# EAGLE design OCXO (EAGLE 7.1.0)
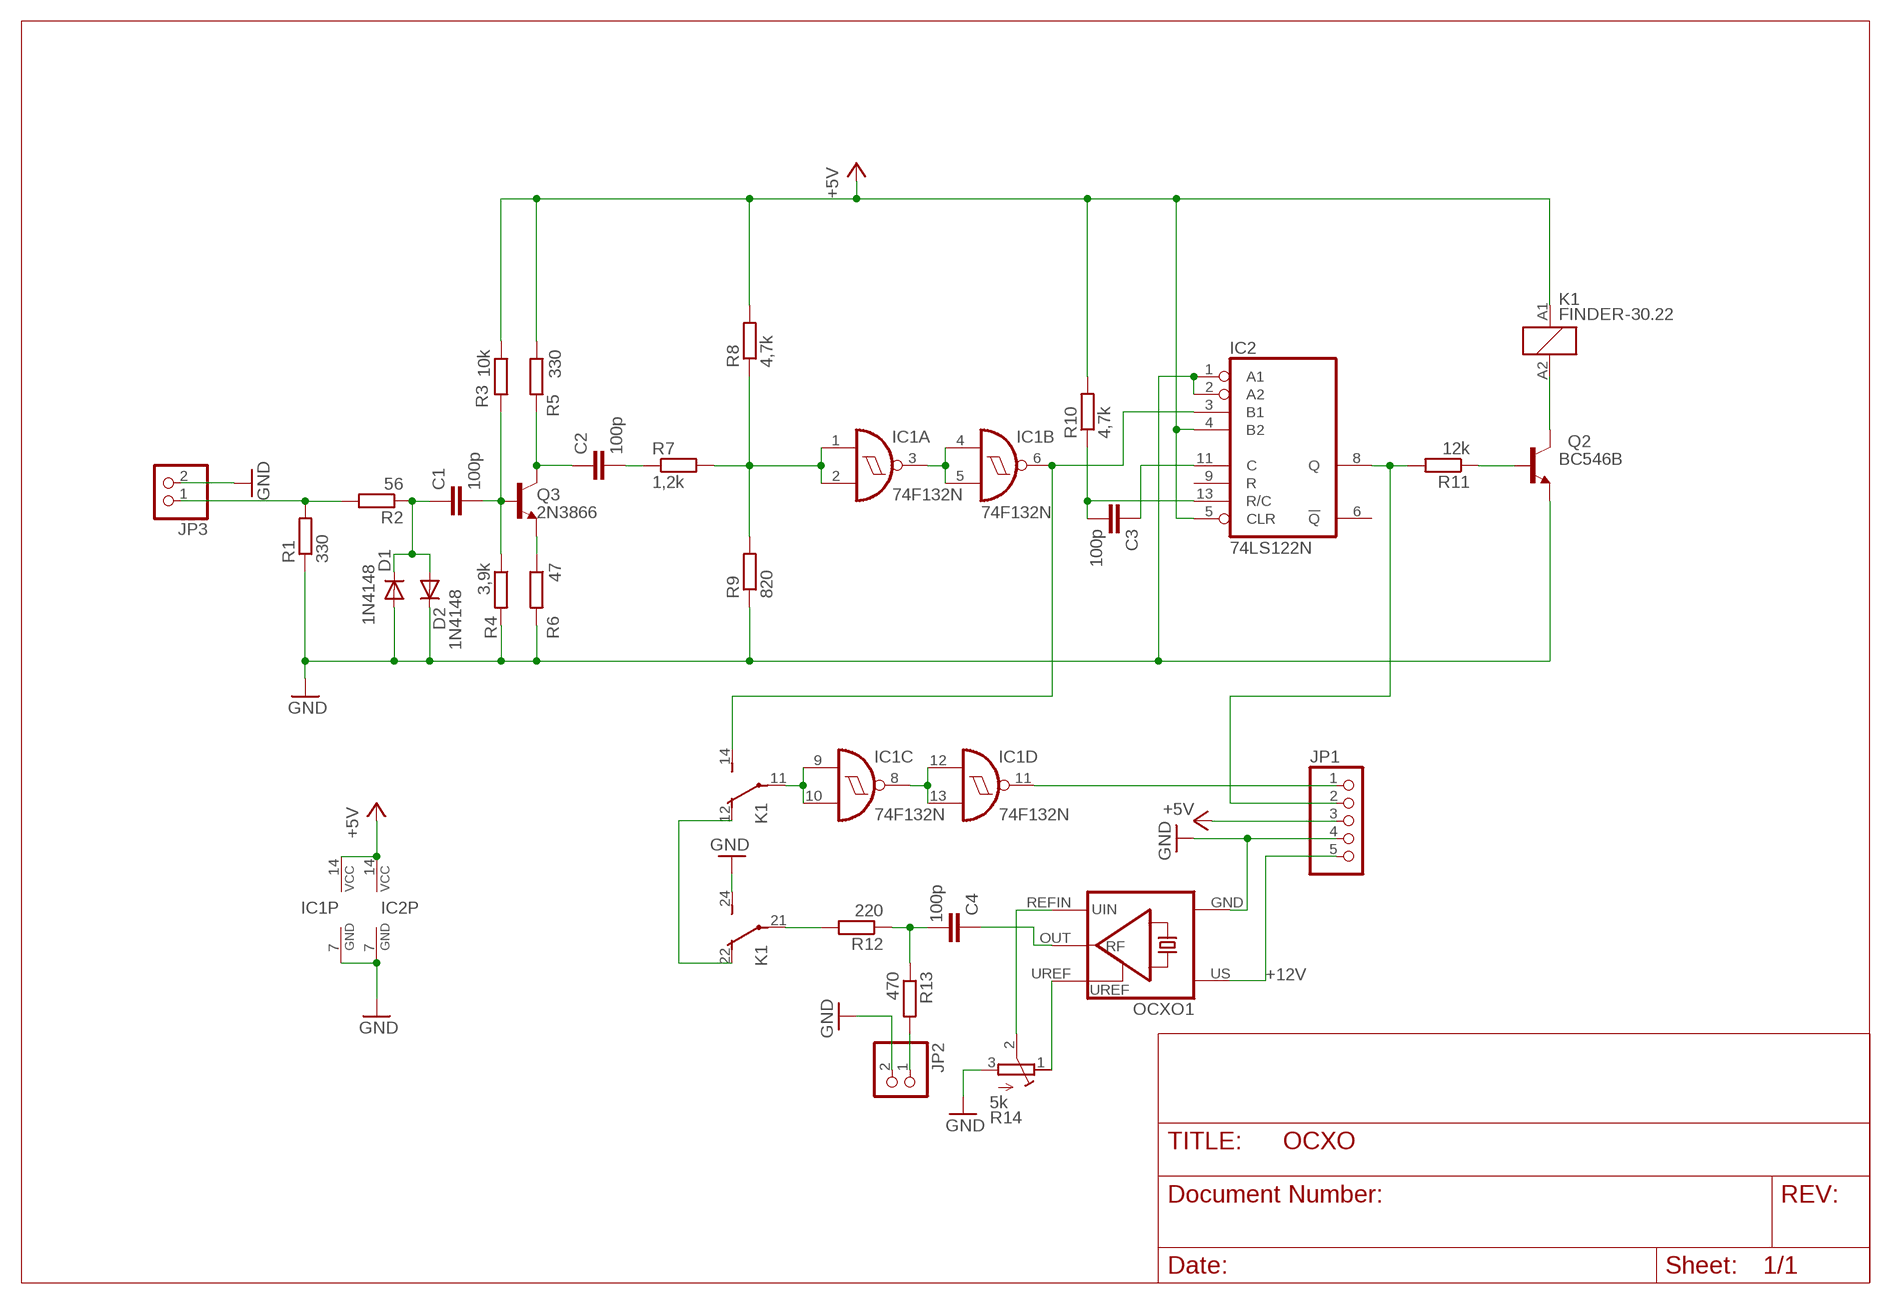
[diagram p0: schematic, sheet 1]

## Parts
C1  100p  C-EU025-024X044  [C025-024X044]
C2  100p  C-EU025-024X044  [C025-024X044]
C3  100p  C-EU025-024X044  [C025-024X044]
C4  100p  C-EU025-024X044  [C025-024X044]
D1  1N4148  1N4148DO35-7  [DO35-7]
D2  1N4148  1N4148DO35-7  [DO35-7]
IC1  74F132N  74S132N  [DIL14]
IC2  74LS122N  [DIL14]
JP1  PINHD-1X05_2.54-90°  [1X05/90]
JP2  PINHD-1X02_2.54  [1X02]
JP3  PINHD-1X02_2.54  [1X02]
K1  FINDER-30.22  [FINDER-30.22]
OCXO1  OCXO_MV197  [OCXO_MV197]
Q2  BC546B  [TO92-EBC]
Q3  2N3866  BC140-10  [TO39]
R1  330  WIDERSTAND_10  [207.10]
R2  56  WIDERSTAND_10  [207.10]
R3  10k  WIDERSTAND_10  [207.10]
R4  3,9k  WIDERSTAND_10  [207.10]
R5  330  WIDERSTAND_10  [207.10]
R6  47  WIDERSTAND_10  [207.10]
R7  1,2k  WIDERSTAND_10  [207.10]
R8  4,7k  WIDERSTAND_10  [207.10]
R9  820  WIDERSTAND_10  [207.10]
R10  4,7k  WIDERSTAND_10  [207.10]
R11  12k  WIDERSTAND_10  [207.10]
R12  220  WIDERSTAND_10  [207.10]
R13  470  WIDERSTAND_10  [207.10]
R14  5k  R-TRIMM43P  [RTRIM43P]

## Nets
+5V: IC1.14(P:VCC) IC2.4(B2) IC2.5(CLR) IC2.14(VCC) JP1.3 K1.A1 R3.1 R5.1 R8.2 R10.2
+12V: JP1.5 OCXO1.US
GND: D1.A D2.C IC1.7(P:GND) IC2.1(A1) IC2.2(A2) IC2.7(GND) JP1.4 JP2.2 JP3.2 K1.24(-2:S) OCXO1.GND Q2.E R1.1 R4.2 R6.2 R9.1 R14.3(E)
N$1: JP3.1 R1.2 R2.2
N$2: C1.1 D1.C D2.A R2.1
N$3: C3.1 IC2.11(C)
N$4: C1.2 Q3.2(B) R3.2 R4.1
N$5: Q3.1(E) R6.1
N$6: C2.1 Q3.3(C) R5.2
N$7: C2.2 R7.1
N$8: IC1.1(A:I0) IC1.2(A:I1) R7.2 R8.1 R9.2
N$9: IC1.3(A:O) IC1.4(B:I0) IC1.5(B:I1)
N$10: IC1.6(B:O) IC2.3(B1) K1.14(-1:S)
N$11: IC2.8(Q) JP1.2 R11.2
N$12: Q2.B R11.1
N$13: K1.A2 Q2.C
N$14: C3.2 IC2.13(R/C) R10.1
N$15: IC1.8(C:O) IC1.12(D:I0) IC1.13(D:I1)
N$16: IC1.11(D:O) JP1.1
N$17: IC1.9(C:I0) IC1.10(C:I1) K1.11(-1:P)
N$18: K1.12(-1:O) K1.22(-2:O)
N$19: K1.21(-2:P) R12.2
N$20: C4.2 R12.1 R13.1
N$21: JP2.1 R13.2
N$22: C4.1 OCXO1.OUT(RF)
N$23: OCXO1.REFIN(UIN) R14.2(S)
N$24: OCXO1.UREF R14.1(A)
Unconnected: IC2.6(!Q) IC2.9(R)

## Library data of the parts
C1-C4 = rcl:C-EU: CAPACITOR, European symbol
D1 D2 = diode:1N4148: DIODE
IC1 = 74xx-eu:74*132: Quad 2-input NAND schmitt trigger
IC2 = 74xx-eu:74*122: Retriggerable monostable MULTIVIBRATOR
JP1 = pinhead-2:PINHD-1X05: PIN HEADER
JP2 JP3 = pinhead-2:PINHD-1X02: PIN HEADER
K1 = relay:FINDER-30.22: SUBMINIATURE DIL-RELAIS FINDER 30.22.9.024.0000 Kontakt max. AC - 125V Distributor: Farnell Bestell Nr.: 1217371 Source: http://www.farnell.com/datasheets/87634.pdf
OCXO1 = 1Eigene:OCXO_MV197
Q2 = transistor-npn:BC546*: NPN Transistor
Q3 = transistor-npn:BC140-10: NPN Transistor
R1-R13 = 1Eigene:WIDERSTAND_10
R14 = rcl:R-TRIMM: Trimm resistor

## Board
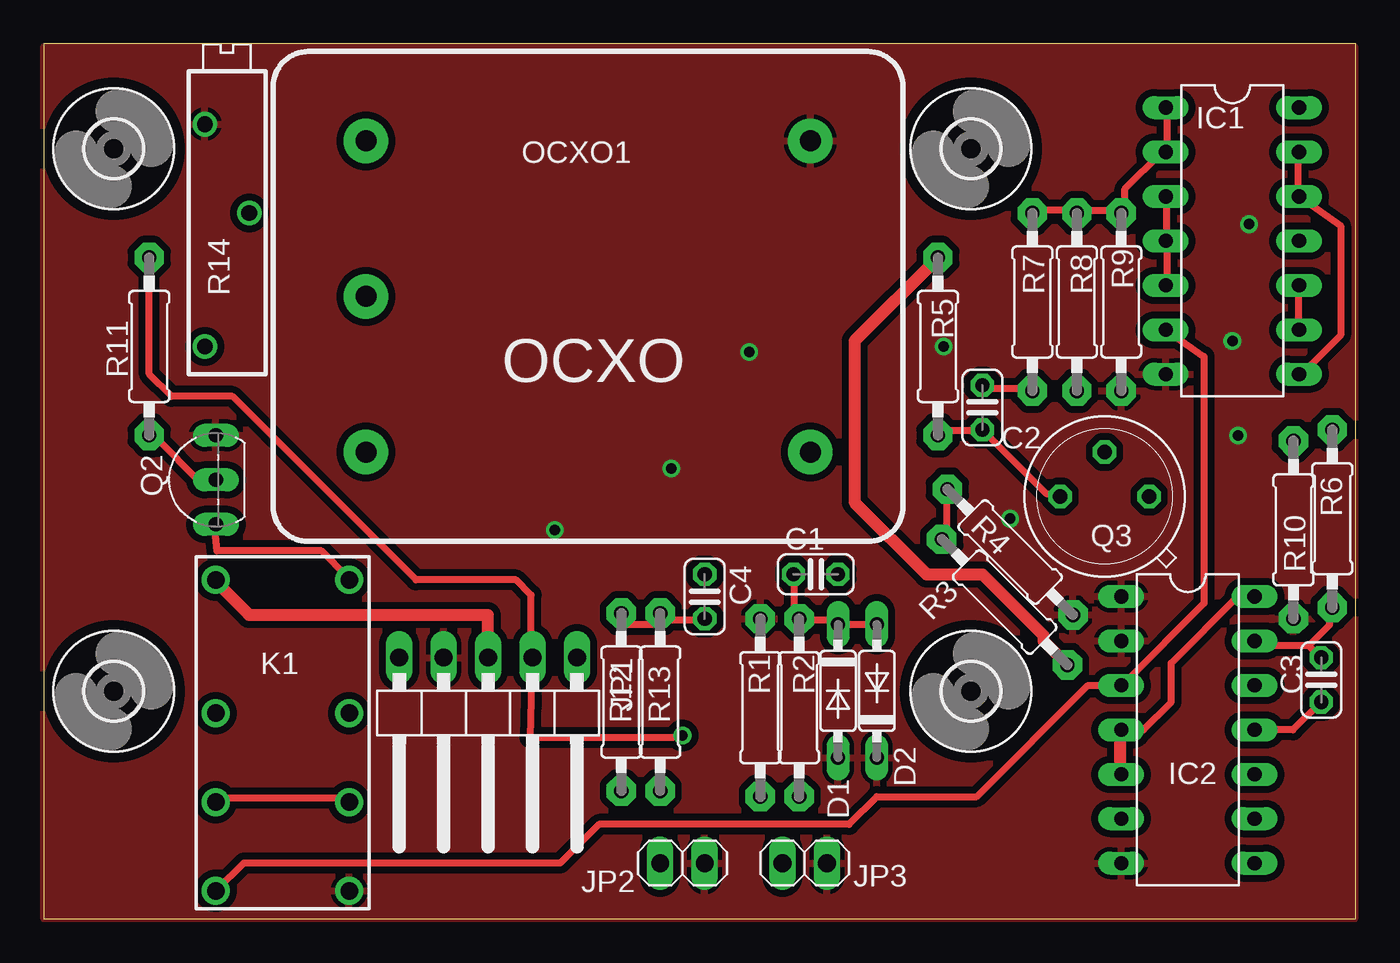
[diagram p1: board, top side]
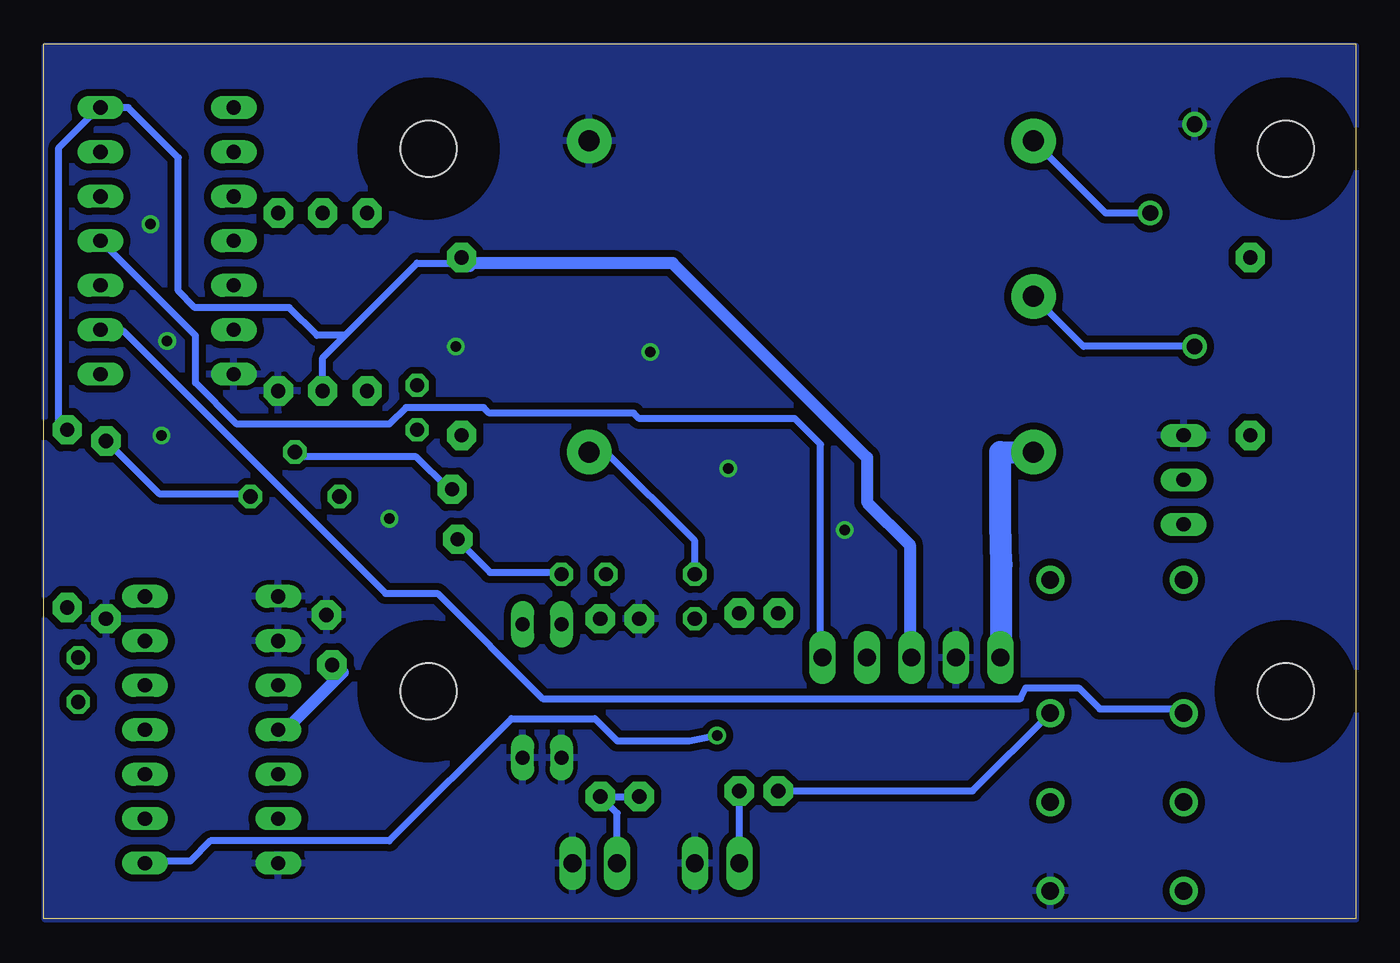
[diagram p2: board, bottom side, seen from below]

Size 75 x 50 mm. Coordinates in mm from the lower left corner, seen from the top.
Outline: 0,0 75,0 75,50 0,50 0,0
Copper layers (1*16): Top 0.035mm / dielectric 1.5mm / Bottom 0.035mm
Design rules "default *": minimum track width 0.4mm, minimum drill 0.6mm, track to track 0.4mm, track to pad 0.4mm, pad to pad 0.4mm, via to via 0.4mm, smd to smd 0.2mm, copper to edge 0mil, drill to drill 8mil, minimum pad ring 10mil, minimum via ring 8mil, stop-mask expansion 4mil, vias tented up to drill 0mil, thermal gap 10mil

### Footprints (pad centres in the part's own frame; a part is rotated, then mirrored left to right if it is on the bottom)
C025-024X044 = drill 0.813 octagon: 1 -1.27,0; 2 1.27,0
DO35-7 = drill 0.813 long: A 3.81,0; C -3.81,0
DIL14 = drill 0.813 long: 1 -7.62,-3.81; 2 -5.08,-3.81; 3 -2.54,-3.81; 4 0,-3.81; 5 2.54,-3.81; 6 5.08,-3.81; 7 7.62,-3.81; 8 7.62,3.81; 9 5.08,3.81; 10 2.54,3.81; 11 0,3.81; 12 -2.54,3.81; 13 -5.08,3.81; 14 -7.62,3.81
1X05/90 = drill 1.016 long: 1 -5.08,-3.81; 2 -2.54,-3.81; 3 0,-3.81; 4 2.54,-3.81; 5 5.08,-3.81
1X02 = drill 1.016 long: 1 -1.27,0; 2 1.27,0
FINDER-30.22 = drill 1 pad 1.6: 11 -1.27,-3.81; 12 3.81,-3.81; 14 8.89,-3.81; 21 -1.27,3.81; 22 3.81,3.81; 24 8.89,3.81; A1 -8.89,-3.81; A2 -8.89,3.81
OCXO_MV197 = drill 1.2 pad 2.54: GND 12.7,8.89; OUT 12.7,-8.89; REFIN -12.7,8.89; UREF -12.7,0; US -12.7,-8.89
TO92-EBC = drill 0.813 long: B 0,-1.27; C -2.54,-1.27; E 2.54,-1.27
TO39 = drill 0.813 octagon: 1 0,-2.54; 2 2.54,0; 3 0,2.54
207.10 = drill 0.813 pad 1.676 octagon: 1 -5.08,0; 2 5.08,0
RTRIM43P = drill 0.9: 1 -7.62,1.27; 2 0,-1.27; 3 5.08,1.27
3,2 = hole 3.2: 0,0

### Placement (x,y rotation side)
C1  44.13,19.68 0 top
C2  53.66,29.21 90 top
C3  73.03,13.65 90 top
C4  37.78,18.41 270 top
D1  45.4,13.02 270 top
D2  47.62,13.02 90 top
IC1  67.94,38.73 270 top
IC2  65.41,10.79 270 top
JP1  25.4,11.11 180 top
JP2  36.51,3.17 0 top
JP3  43.5,3.17 0 top
K1  13.65,10.48 270 top
OCXO1  31.11,35.56 0 top
Q2  8.57,25.08 90 top
Q3  60.64,24.13 90 top
R1  40.96,12.06 270 top
R2  43.18,12.06 270 top
R3  54.93,18.1 135 top
R4  55.24,20.95 315 top
R5  51.12,32.7 270 top
R6  71.44,22.23 270 top
R7  56.52,35.24 90 top
R8  59.05,35.24 270 top
R9  61.59,35.24 90 top
R10  73.66,22.86 90 top
R11  6.03,32.7 90 top
R12  33.02,12.38 270 top
R13  35.24,12.38 270 top
R14  10.48,40.32 90 top
U$1  [3,2]  4,44 0 top
U$2  [3,2]  53,44 0 top
U$3  [3,2]  4,13 0 top
U$4  [3,2]  53,13 0 top

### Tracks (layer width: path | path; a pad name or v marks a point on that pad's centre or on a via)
+5V
  Top 0.4: 9.9,19.2 K1.A1 | 61.5,8.4 IC2.5 | 61.5,10.5 IC2.4 61.5,10.8 62.87,10.8 64.45,12.38 64.45,14.61 68.26,18.41 IC2.14 69,18.3 | JP1.3 25.6,15.2 25.33,15.21
  Top 0.7: 25.32,14.88 25.33,15.21 25.38,17.36 11.73,17.36 9.9,19.2 | 61.5,10.5 61.5,8.4 | R5.1 46.35,33.02 46.35,23.81 50.48,19.68 53.66,19.68 57.15,16.19 57.15,15.88 R3.1
  Bottom 0.4: 58.53,14.42 R3.1 | 61.5,10.48 IC2.4 | 25.5,15 25.32,14.88 | R8.2 59.05,32.07 57.78,33.34 | 57.78,33.34 53.66,37.47 51.44,37.47 R5.1 | R10.2 74.14,28.2 74.14,44.06 72,46.2 IC1.14 70.17,46.35 67.31,43.5 67.31,35.88 66.36,34.92 60.96,34.92 59.37,33.34 57.78,33.34 | JP1.3 25.6,15.2 25.5,15.2
  Bottom 0.7: 58.53,14.42 57.9,14.08 61.5,10.48 | 25.5,15 25.5,15.2 25.5,21.37 27.94,23.81 27.94,26.35 39.05,37.47 50.48,37.47 50.64,37.31 R5.1
+12V
  Bottom 0.4: JP1.5 20.4,15.2 20.25,15.2
  Bottom 1.27: 20.25,14.88 20.25,15.2 20.25,20.25 20.32,22.54 20.32,26.67 OCXO1.US
GND  (via drill 0.6)
  other vias: 67.94,33.02 68.26,27.62 40.32,32.38 51.44,32.7 29.21,22.23 55.24,22.86 68.9,39.69 35.88,25.72
  pour Bottom: 0,49.85 74.93,49.85 74.93,0 0,0 0,49.53
  pour Top: 0,0 0,49.85 74.93,49.85 74.93,0
N$1
  Bottom 0.4: JP3.1 42.23,6.03 R2.2 R1.2
N$2
  Top 0.4: D2.A 47.4,16.8 45.6,16.8 D1.C 45.3,17.1 43.2,17.1 R2.1 42.9,17.4 42.9,19.5 C1.1
N$3
  Top 0.4: IC2.11 69.3,10.8 71.4,10.8 72.9,12.3 C3.1
N$4
  Top 0.4: R3.2 51.6,21.9 51.6,24.3 R4.1
  Bottom 0.4: C1.2 45.6,19.8 49.5,19.8 51.3,21.6 R3.2 | Q3.2 60.6,26.4 53.7,26.4 51.9,24.6 R4.1
N$5
  Bottom 0.4: Q3.1 63.3,24.3 68.4,24.3 71.4,27.3 R6.1
N$6
  Top 0.4: Q3.3 57.9,24.3 57.3,24.3 53.7,27.9 C2.1 53.4,27.9 51.3,27.9 R5.2
N$7
  Top 0.4: C2.2 53.7,30.3 56.4,30.3 R7.1
N$8
  Top 0.4: IC1.1 64.2,46.2 64.2,44.1 IC1.2 63.9,43.8 61.8,41.7 61.8,40.5 R9.2 61.5,40.5 59.1,40.5 R8.1 58.8,40.5 56.7,40.5 R7.2
N$9
  Top 0.4: IC1.5 64.2,36.3 64.2,38.7 IC1.4 64.2,39 64.2,41.1 IC1.3
N$10
  Top 0.4: IC2.3 61.8,13.5 66.32,18.02 66.32,32.12 64.2,33.6 IC1.6 | 9.9,1.5 K1.14 11.43,3.17 29.53,3.17 31.75,5.4 46.04,5.4 47.62,6.99 53.34,6.99 59.69,13.34 IC2.3 | 61.5,13.2 IC2.3
N$11  (via drill 0.6)
  Top 0.4: v36.51,10.48 35.99,10.36 27.8,10.36 27.9,14.7 27.86,14.88 27.86,15.2 | 27.86,15.2 27.86,18.49 26.99,19.37 21.27,19.37 10.79,29.84 7.3,29.84 6.03,31.11 R11.2 | JP1.2 28,15.2 27.86,15.2
  Bottom 0.4: IC2.8 69,3.3 66.62,3.3 65.47,4.45 55.24,4.45 48.26,11.43 43.5,11.43 42.23,10.16 38.1,10.16 v36.51,10.48
N$12
  Top 0.4: Q2.B 9.32,24.95 9,24.9 6.3,27.6 R11.1
N$13
  Top 0.4: Q2.C 9.76,22.43 9.9,21.02 15.88,21.02 17.4,19.5 K1.A2
N$14
  Top 0.4: 72.3,15.6 69.3,15.6 IC2.13 | 72.3,15.6 72.9,15 C3.2 | 72.3,15.6 73.5,16.8 73.5,17.7 R10.1
N$15
  Top 0.4: IC1.8 72,31.2 74.14,33.34 74.14,39.6 72,41.1 IC1.12 71.7,41.4 71.7,43.8 IC1.13
N$16
  Bottom 0.4: IC1.11 71.7,38.7 66.32,33.32 66.32,30.62 63.96,28.26 55.24,28.26 54.29,29.21 49.85,29.21 49.53,28.89 41.27,28.89 40.96,28.57 32.07,28.57 30.6,27.11 30.6,15 30.41,14.88 30.4,14.8 JP1.1
N$17
  Top 0.4: IC1.9 71.7,33.9 71.7,36 IC1.10
  Bottom 0.4: K1.11 9.9,12 14.63,12 15.83,13.2 18.86,13.2 19.16,12.58 46.48,12.58 52.5,18.6 55.47,18.6 70.47,33.6 71.7,33.6 IC1.9
N$18
  Top 0.4: K1.12 9.9,6.9 17.4,6.9 K1.22
N$19
  Bottom 0.4: R12.2 21.91,7.3 K1.21
N$20
  Top 0.4: C4.2 37.5,17.1 35.4,17.1 R13.1 35.1,16.8 33.3,16.8 R12.1
N$21
  Bottom 0.4: JP2.1 R13.2
N$22
  Bottom 0.4: C4.1 37.78,21.59 42.86,26.67 OCXO1.OUT
N$23
  Bottom 0.4: R14.2 14.29,40.32 OCXO1.REFIN
N$24
  Bottom 0.4: R14.1 15.56,32.7 OCXO1.UREF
